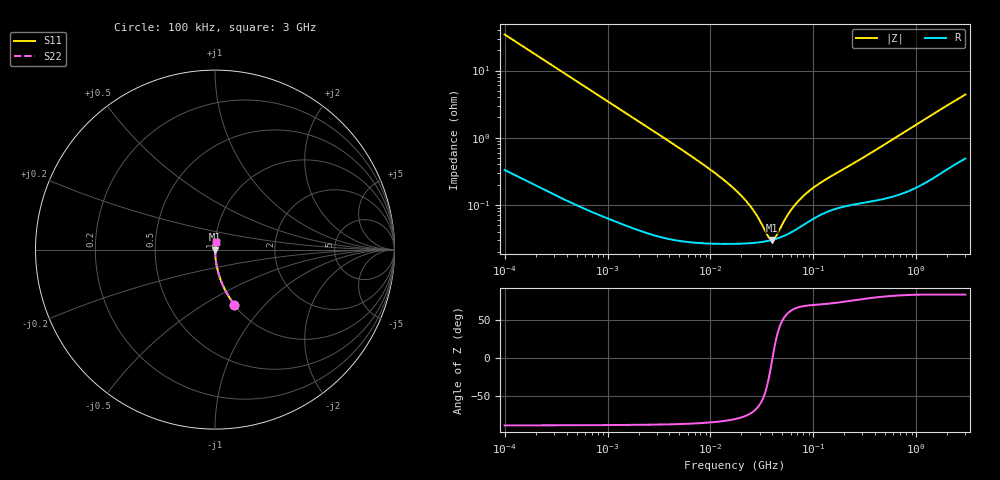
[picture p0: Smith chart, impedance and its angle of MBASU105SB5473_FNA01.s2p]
! MBASU105SB5473_FNA01  S-PARAMETER MODEL  ( Standard Model )
! Model Generated by TAIYO YUDEN Corporation (http://www.ty-top.com)
! Version 1.0
! TAIYO YUDEN Control No. 220601
! Copyright(c) 2014 TAIYO YUDEN CO.,LTD. All Rights Reserved.
! Product Description (link to TY-COMPAS)
! https://ds.yuden.co.jp/TYCOMPAS/or/detail?pn=MBASU105SB5473KFNA01&u=M
! Products Name : Multilayer Ceramic Capacitors
! Characteristics :
!  Capacitance : 0.047 [uF] , Rated Voltage : 50 [V] , TCC : X5R
!  Case Size : 1.0 x 0.5 / 0.039 x 0.02 [mm/inch] , Thickness : 0.5 / 0.02 [mm/inch]
!  (Conditions: Temperature = 25 [degC] , DC Bias Voltage = 0 [V])
! External Node Assignments :
!  1  o---| |---o  2
! GND o---------o GND
! Frequency Range : 100kHz  -  3GHz  [ 401 STEP ]
# MHZ S RI R 50
! Freq[MHz].  S11 Real  S11 Imag  S21 Real  S21 Imag  S12 Real  S12 Imag  S22 Real  S22 Imag
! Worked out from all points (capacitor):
!   401 points, 100 kHz to 3 GHz, reference 50 ohm
!   read as one part in series: C = 46.1 nF near 105.3 kHz
!   lowest |Z| = 30 mohm at 39.51 MHz (marker M1)
!   series resonance near 40.12 MHz, so ESL is about 340 pH
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0.1  0.1086 -0.3063  0.8914 0.3063  0.8914 0.3063  0.1086 -0.3063
0.147195  0.0543 -0.2215  0.9457 0.2215  0.9457 0.2215  0.0543 -0.2215
0.228123  0.0242 -0.148  0.9758 0.148  0.9758 0.148  0.0242 -0.148
0.562235  0.00473 -0.0617  0.9953 0.0617  0.9953 0.0617  0.00473 -0.0617
3.161081  0.000458 -0.0111  0.9995 0.0111  0.9995 0.0111  0.000458 -0.0111
9.574722  0.000277 -0.00349  0.9997 0.00349  0.9997 0.00349  0.000277 -0.00349
13.38544  0.000267 -0.00236  0.9997 0.00236  0.9997 0.00236  0.000267 -0.00236
17.7727  0.000265 -0.00161  0.9997 0.00161  0.9997 0.00161  0.000265 -0.00161
21.84217  0.000267 -0.00114  0.9997 0.00114  0.9997 0.00114  0.000267 -0.00114
25.49486  0.00027 -0.000832  0.9997 0.000832  0.9997 0.000832  0.00027 -0.000832
29.00125  0.000275 -0.000586  0.9997 0.000586  0.9997 0.000586  0.000275 -0.000586
36.57227  0.000291 -0.000164  0.9997 0.000164  0.9997 0.000164  0.000291 -0.000164
39.51212  0.000299 -2.71e-05  0.9997 2.71e-05  0.9997 2.71e-05  0.000299 -2.71e-05
41.60216  0.000305 6.43e-05  0.9997 -6.43e-05  0.9997 -6.43e-05  0.000305 6.43e-05
43.80277  0.000313 0.000156  0.9997 -0.000156  0.9997 -0.000156  0.000313 0.000156
53.83243  0.000354 0.000524  0.9996 -0.000524  0.9996 -0.000524  0.000354 0.000524
64.47533  0.000409 0.000854  0.9996 -0.000854  0.9996 -0.000854  0.000409 0.000854
77.22239  0.000485 0.00119  0.9995 -0.00119  0.9995 -0.00119  0.000485 0.00119
97.38194  0.000607 0.00164  0.9994 -0.00164  0.9994 -0.00164  0.000607 0.00164
132.6759  0.000776 0.00227  0.9992 -0.00227  0.9992 -0.00227  0.000776 0.00227
547.5153  0.00136 0.00866  0.9986 -0.00866  0.9986 -0.00866  0.00136 0.00866
3000  0.00675 0.0432  0.9933 -0.0432  0.9933 -0.0432  0.00675 0.0432
